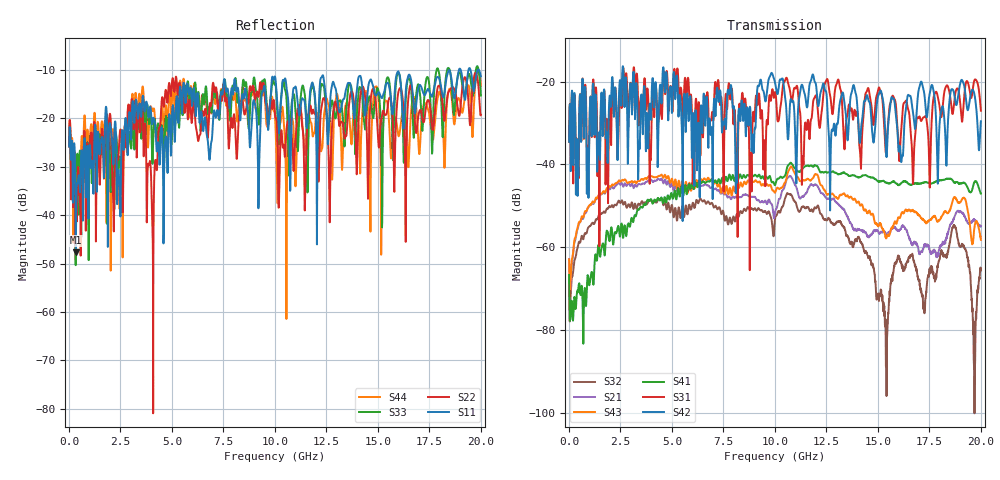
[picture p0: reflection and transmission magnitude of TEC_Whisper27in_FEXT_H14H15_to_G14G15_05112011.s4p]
! Tyco Electronics
! H14H15-G14G15_FEXT
!! PART DESCRIPTION: Whisper 27in Megtron 6 VLP-HVLP-VLP Channel Model, bulkhead 2.4mm test pts
!! MODEL DESCRIPTION: System 4-port S-parameter
!! MODEL STATUS: Measured
!! MODEL GEOMETRY: Channel Model
!! MODEL FREQUENCY RANGE: DC to 20.000 GHz in 10.000 MHz frequency steps
!! MODEL EDGE RATE LIMITATION: 25.00 ps (Using conservative 0.5/Fmax rule of thumb)
!! TIME-DOMAIN TRANSFORM CAUTIONS:
!! 1.) Do not simulate transient edge rates faster than the number listed above.  Edge rates faster than this number
!!  contain significant spectral content at frequencies above the model's highest frequency.
!! 2.) Even when simulating edge rates that are slower than the number listed above, be aware that the best time
!!  resolution possible with a direct iFFT is (1 / 2Fmax).  As a result, time resolution is typically not adequate
!!  for most time-domain simulations unless tricks such as windowing are used to minimize leakage and aliasing.
!! 3.) Because the model has a uniform frequency step, a direct iFFT will result in an impulse that that has a time
!!  length given by either (1 / Fstep) or (1 / 2Fstep), depending on the transform being used.  Care has been taken
!!  in selecting the frequency step to ensure a settled impulse response for the model.  Therefore, convolution with
!!  the model's impulse response should present no issues.  However, if directly concatenating s-parameter models
!!  in the frequency domain a user must either interpolate necessary interim frequencies or complete impulse response
!!  zero-padding.  Impulse response zero-padding is more difficult, but more accurate.
!! PORT DEFINITIONS:
!! Port  1  ----->  Side A  H14  G14  Side B  <-----  Port  2
!! Port  3  ----->  Side A  H15  G15  Side B  <-----  Port  4
! Point-to-Point link (differential)  !
! Connectors:  !
!  1: STRADA Whisper  !
! Materials:  !
!  Backplane: Megtron-6 HVLP  !
!  Daughtercard: Megtron-6 VLP  !
! Stack-up:  !
!  Backplane: 20 layers, 200mil thick  !
!  Daughtercard: 14 layers, 110mil thick  !
! Trace Length:  !
!  Backplane: 17in  !
!  Daightercards: 5in  !
! Trace Width:  !
!  Backplane: 8-13-8 mils  !
!  Daughtercards: 6-9-6 mils  !
! Geometry:  !
!  Backplane: Stripline  !
!  Daughtercards: Stripline  !
! Freq. Range: 0 GHz - 20 GHz  !
! Note1: non-mixed-mode s-parameters  !
! Note2: channel includes 2.4mm test points  !
! Created Wed May 11 14:44:54 2011
! 4 Port Network Data from SP1.SP block
! freq  magS11  angS11  magS12  angS12  magS13  angS13  magS14  angS14
!  magS21  angS21  magS22  angS22  magS23  angS23  magS24  angS24
!  magS31  angS31  magS32  angS32  magS33  angS33  magS34  angS34
!  magS41  angS41  magS42  angS42  magS43  angS43  magS44  angS44
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# hz S ma R 50
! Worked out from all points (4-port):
!   2000 points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, 10 MHz to 20 GHz, reference 50 ohm
!   strongest paths, dB at 10 MHz, 5.01 GHz, 10.01 GHz, 15.01 GHz, 20 GHz:
!     S42: -34.5, -27.4, -20.3, -23.4, -29.5
!     S31: -34.6, -26.0, -22.5, -22.0, -27.0
!     S41: -66.7, -47.5, -45.0, -44.1, -47.1
!     S43: -62.9, -43.5, -46.8, -54.7, -58.2
!     S21: -62.9, -44.7, -51.6, -56.2, -55.0
!     S32: -67.1, -50.0, -53.1, -71.2, -65.2
!   lowest |S11| = -47.7 dB at 340 MHz (marker M1), VSWR 1.01, Z = 50.2 + j0.351 ohm
!   |S11| at or under -10 dB: start of sweep to 18.94 GHz; 19.01 GHz to 19.4 GHz (390.9 MHz wide, 2.03 % of centre); 19.49 GHz to end of sweep
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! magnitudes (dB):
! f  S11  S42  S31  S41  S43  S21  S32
! 10 MHz  -25.9  -34.5  -34.6  -66.7  -62.9  -62.9  -67.1
! 340 MHz  -47.7  -47.3  -41.4  -74.1  -57.1  -57.5  -62.1
! 6.4 GHz  -19.0  -26.5  -32.4  -44.5  -43.5  -45.1  -48.3
! 13.15 GHz  -18.8  -25.1  -21.2  -42.3  -47.4  -50.0  -53.7
! 15.42 GHz  -12.8  -38.2  -34.9  -44.5  -57.6  -56.9  -96.0
! 18.68 GHz  -15.7  -22.4  -26.0  -44.2  -48.1  -53.3  -54.7
! 20 GHz  -11.4  -29.5  -27.0  -47.1  -58.2  -55.0  -65.2
